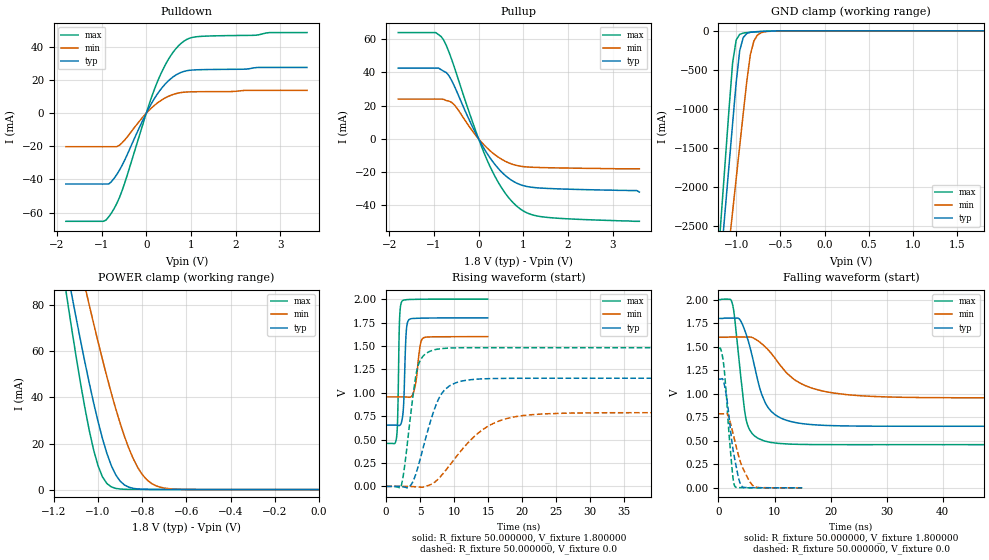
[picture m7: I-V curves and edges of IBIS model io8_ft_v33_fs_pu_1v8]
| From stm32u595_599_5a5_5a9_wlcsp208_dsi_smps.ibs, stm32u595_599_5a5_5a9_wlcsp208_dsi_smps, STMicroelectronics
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|   Model io8_ft_v33_fs_pu_1v8
[Model]  io8_ft_v33_fs_pu_1v8
Model_type I/O
Polarity   Non-Inverting
Enable   Active-Low
Vinl =   0.540000V
Vinh =   1.260000V
Vmeas =  0.900000V
Cref =   50.000000pF
Rref =   100.000000M
Vref =   0.0V
C_comp   3.087500pF   3.086600pF   3.135700pF
[Temperature Range]   25.000000   0.140000k   -40.000000
[Pullup Reference]   1.800000V   1.600000V   2.000000V
[Pulldown Reference]   0.0V   0.0V   0.0V
[POWER Clamp Reference]   1.800000V   1.600000V   2.000000V
[GND Clamp Reference]   0.0V   0.0V   0.0V
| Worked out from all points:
|   slope of the pulldown table from 0 to 0.27 V, typ, clamps not added: 21.7 ohm
|   slope of the pullup table from 0 to 0.27 V, typ, clamps not added: 22.6 ohm
|   GND clamp passes 1 mA (typ) near -0.51 V on its own axis
|   POWER clamp passes 1 mA (typ) near -0.86 V on its own axis
|   rising waveform, R_fixture 50.000000, V_fixture 1.800000: 20-80 % time 316ps typ, 629ps min, 228ps max; typ from 0.655 V to 1.8 V
|   rising waveform, R_fixture 50.000000, V_fixture 0.0: 20-80 % time 2.89ns typ, 6.11ns min, 1.52ns max; typ from 0.001 V to 1.16 V
|   falling waveform, R_fixture 50.000000, V_fixture 1.800000: 20-80 % time 3.27ns typ, 6.78ns min, 1.71ns max; typ from 1.8 V to 0.655 V
|   falling waveform, R_fixture 50.000000, V_fixture 0.0: 20-80 % time 1.6ns typ, 2.38ns min, 1.14ns max; typ from 1.16 V to 0.001 V
[Pulldown]
|Voltage   I(typ)   I(min)   I(max)
-1.8V     -42.74mA   -20.21mA   -65.25mA
-960mV    -42.74mA   -20.21mA   -65.25mA
-780mV    -41.3mA    -20.21mA   -60.25mA
-660mV    -37mA      -20.2mA    -54.5mA
-540mV    -31.39mA   -17.82mA   -46.65mA
0V        0A         0A         0A
240mV     11.28mA    6.002mA    18.38mA
480mV     19.17mA    10.02mA    31.83mA
780mV     24.67mA    12.5mA     42.21mA
960mV     25.9mA     12.9mA     45.21mA
1.2V      26.29mA    13.01mA    46.37mA
3.6V      27.66mA    13.81mA    48.71mA
[Pullup]
|Voltage   I(typ)   I(min)   I(max)
-1.8V     42.57mA    23.91mA    63.93mA
-960mV    42.57mA    23.91mA    63.93mA
-780mV    40.65mA    23.73mA    59.33mA
-660mV    37.77mA    22.64mA    51.97mA
-540mV    31.57mA    20.34mA    42.81mA
-120mV    6.338mA    4.065mA    8.965mA
180mV     -8.368mA   -5.234mA   -12.14mA
540mV     -20.62mA   -12.68mA   -30.5mA
900mV     -27.22mA   -16.28mA   -41.49mA
1.14V     -28.94mA   -17mA      -45.14mA
1.5V      -29.77mA   -17.34mA   -47.14mA
3.6V      -32mA      -18mA      -49.6mA
[GND_clamp]
|Voltage   I(typ)   I(min)   I(max)
-1.8V     -9.707A    -9.942A    -9.774A
-1.2V     -3.309A    -4.006A    -2.864A
-1.16V    -2.777A    -3.584A    -2.239A
-1.12V    -2.246A    -3.162A    -1.614A
-1.04V    -1.186A    -2.319A    -408.6mA
-1V       -663.9mA   -1.898A    -117.8mA
-960mV    -254mA     -1.478A    -45.14mA
-920mV    -86.03mA   -1.06A     -28.58mA
-840mV    -19.12mA   -308.9mA   -18.74mA
-800mV    -13.39mA   -130.8mA   -15.31mA
-720mV    -7.948mA   -25.37mA   -9.381mA
1.8V      0A         14.97nA    0A
[POWER_clamp]
|Voltage   I(typ)   I(min)   I(max)
-1.8V     470.9mA    433.7mA    554.6mA
-1.14V    95.29mA    122.7mA    82.89mA
-1.12V    85mA       114mA      70.34mA
-1.06V    55.55mA    88.43mA    35.74mA
-1.04V    46.38mA    80.17mA    25.83mA
-1V       29.54mA    64.14mA    10.37mA
-940mV    10.43mA    41.88mA    1.179mA
-900mV    3.662mA    28.79mA    252.8uA
-840mV    528.6uA    13.26mA    97.33uA
-800mV    159uA      6.55mA     88.9uA
-740mV    60.12uA    1.751mA    70.99uA
0V        0A         18.15nA    0A
[Ramp]
| variable   typ   min   max
dV/dt_r  0.69287/2.88568n   0.47203/6.10466n   0.88855/1.51853n
dV/dt_f  0.68715/3.26967n   0.38638/6.76948n   0.92438/1.71054n
R_load = 50.000000
[Rising Waveform]
R_fixture= 50.000000
V_fixture= 1.800000
V_fixture_min= 1.600000
V_fixture_max= 2.000000
|time   V(typ)   V(min)   V(max)
0s        654.8mV    956mV      459.4mV
1.562ns   654.2mV    956.1mV    542.1mV
1.712ns   653mV      956.1mV    781.1mV
1.982ns   651.6mV    956.1mV    1.795V
2.342ns   711.4mV    956mV      1.978V
2.583ns   887mV      955.8mV    1.989V
2.943ns   1.633V     954.9mV    1.994V
3.333ns   1.778V     952mV      1.996V
5.345ns   1.797V     1.578V     1.999V
14.95ns   1.8V       1.6V       2V
[Rising Waveform]
R_fixture= 50.000000
V_fixture= 0.0
V_fixture_min= 0.0
V_fixture_max= 0.0
|time   V(typ)   V(min)   V(max)
0s        615.9uV    687.1uV    590.9uV
2.242ns   -2.446mV   693.9uV    12.79mV
3.524ns   5.236mV    5.257uV    712.1mV
4.645ns   197mV      -5.238mV   1.276V
7.207ns   843.5mV    48.36mV    1.461V
8.328ns   1.006V     132.3mV    1.473V
10.25ns   1.106V     309.9mV    1.479V
14.41ns   1.149V     615.8mV    1.481V
19.86ns   1.155V     753.6mV    1.481V
79.76ns   1.155V     787.4mV    1.481V
[Falling Waveform]
R_fixture= 50.000000
V_fixture= 1.800000
V_fixture_min= 1.600000
V_fixture_max= 2.000000
|time   V(typ)   V(min)   V(max)
0s        1.8V       1.6V       2V
2.402ns   1.804V     1.603V     1.971V
2.883ns   1.803V     1.603V     1.807V
3.684ns   1.797V     1.603V     1.349V
4.965ns   1.627V     1.602V     716.6mV
6.086ns   1.382V     1.596V     572.5mV
8.168ns   928.5mV    1.507V     498.7mV
13.61ns   695.5mV    1.147V     463.7mV
20.66ns   661mV      1.007V     459.7mV
79.76ns   654.8mV    956mV      459.4mV
[Falling Waveform]
R_fixture= 50.000000
V_fixture= 0.0
V_fixture_min= 0.0
V_fixture_max= 0.0
|time   V(typ)   V(min)   V(max)
0s        1.155V     787.4mV    1.481V
420.4ps   1.155V     787.4mV    1.472V
930.9ps   1.124V     787.3mV    1.308V
1.351ns   999.1mV    792.3mV    1.036V
1.622ns   889.4mV    780.3mV    788mV
2.402ns   487.9mV    626.1mV    214.8mV
2.943ns   292.5mV    491.7mV    13.91mV
4.024ns   26.69mV    256.3mV    2.406mV
6.096ns   2.188mV    26.52mV    1.208mV
14.95ns   615.9uV    687.1uV    590.9uV
